PROGRAM MAIN
VAR
	SafeRun				AT%Q*:BOOL;			// 安全程序运行
	SafeErrAck			AT%Q*:BOOL;			// 安全程序复位
	SafeComErr			AT%I*:BOOL;			// ComErr
	SafeOtherErr		AT%I*:BOOL;			// 其他错误
	SLS_MonStatus		AT%I*:BOOL;			// SLS功能开启信号
	SLS_Status			AT%I*:BOOL;			// 进入SLS监控
	Ch3_Status			AT%I*:BOOL;	
	
	Axis1					: AXIS_REF;
	Axis1_Power				: MC_POWER;
	Axis1_MoveVelo			: MC_MoveVelocity;
	Axis1_Halt				: MC_Halt;
	
	Power_On				: BOOL;
	Override				: LREAL;
	Axis1_MoveVelo_Exc		: BOOL;
	Velocity				: LREAL:=2500.0;
	Axis1_Halt_Exc			: BOOL;
	ErrTest					: BOOL:=False;
END_VAR


IF NOT SLS_MonStatus AND NOT ErrTest THEN 
	Override := 18;
ELSE
	Override := 100;
END_IF

Axis1_Power(
	Axis:= Axis1, 
	Enable:= Power_On, 
	Enable_Positive:= Power_On, 
	Enable_Negative:= Power_On, 
	Override:= Override,  
	Error=> , 
	ErrorID=> );
	
Axis1_MoveVelo(
	Axis:= Axis1, 
	Execute:= Axis1_MoveVelo_Exc, 
	Velocity:= Velocity, 
	Error=> , 
	ErrorID=> );
	
Axis1_Halt(
	Axis:= Axis1, 
	Execute:= Axis1_Halt_Exc, 
	Error=> , 
	ErrorID=> );

END_PROGRAM
